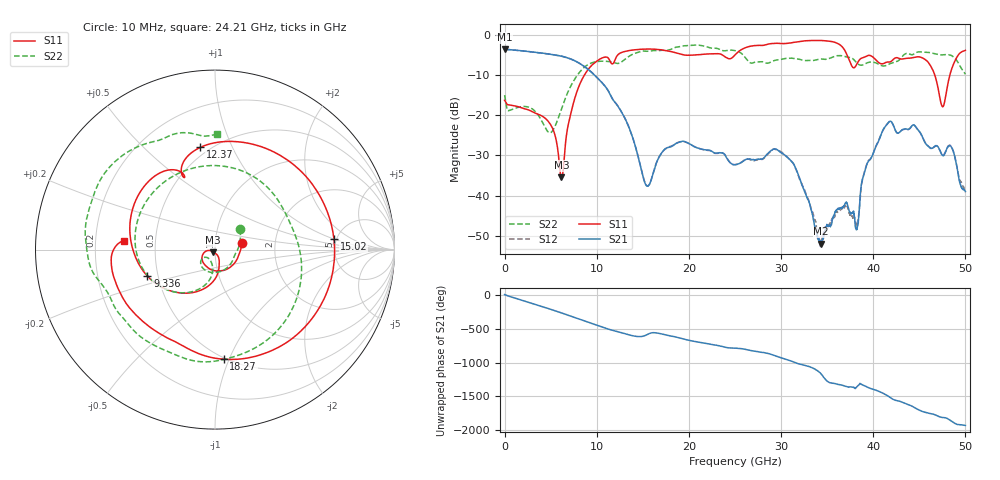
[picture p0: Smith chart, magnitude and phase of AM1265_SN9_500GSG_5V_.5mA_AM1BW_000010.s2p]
!Keysight Technologies,N5245B,MY58422270,A.16.20.02
!Date: Thursday, March 05, 2026 00:26:45
!Correction: S11(C  2-Port  )
!S21(C  2-Port  )
!S12(C  2-Port  )
!S22(C  2-Port  )
!S2P File: Measurements: S11, S21, S12, S22:
# Hz S  dB  R 50
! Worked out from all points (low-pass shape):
!   3201 points, 10 MHz to 50 GHz, reference 50 ohm
!   highest |S21| = -3.57 dB at 10 MHz (marker M1); lowest = -52.0 dB at 34.36 GHz (marker M2)
!   |S21| within 3 dB of the highest: start of sweep to 7.746 GHz
!   lowest |S11| = -35.4 dB at 6.181 GHz (marker M3), VSWR 1.03, Z = 49 - j1.38 ohm
!   |S11| at or under -10 dB: start of sweep to 8.665 GHz; 46.68 GHz to 48.31 GHz (1.63 GHz wide, 3.43 % of centre)
!   |S22| runs from -24.4 to -2.5 dB; largest |S21 - S12| = 0.011
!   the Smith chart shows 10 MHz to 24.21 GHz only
!   S11 on the Smith chart (normalised r, x): 10 MHz: 1.35, +0.11; 9.336 GHz: 0.44, -0.15; 12.37 GHz: 0.45, +0.76; 15.02 GHz: 4.75, +1.02; 18.27 GHz: 0.49, -0.96; 24.21 GHz: 0.32, +0.04
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1e7  -16.26 14.4  -3.57 4.0  -3.60 3.5  -14.99 39.0
2.322038e9  -18.46 -86.1  -4.06 -98.8  -4.06 -98.8  -17.83 -107.5
4.212284e9  -20.39 -135.9  -4.56 -179.3  -4.56 -179.3  -22.20 -145.0
6.180641e9  -35.43 -123.9  -5.29 92.9  -5.30 93.0  -18.45 -96.3
8.352081e9  -11.34 -117.8  -7.38 -10.1  -7.38 -10.0  -8.74 -145.5
9.336259e9  -7.86 -158.5  -9.08 -56.7  -9.06 -56.6  -7.07 178.2
1.107029e10  -5.52 129.4  -13.26 -136.4  -13.26 -136.4  -6.57 97.6
1.23669e10  -4.80 98.2  -17.95 173.1  -17.95 173.1  -7.09 22.5
1.502262e10  -3.54 5.2  -35.25 108.7  -35.11 108.6  -4.00 -99.9
1.667854e10  -3.62 -44.5  -30.79 153.3  -30.76 153.8  -3.91 -141.1
1.827197e10  -4.26 -85.4  -27.54 106.5  -27.49 106.5  -3.37 -166.7
2.420828e10  -5.82 174.5  -31.02 -60.7  -30.94 -60.2  -3.84 88.8
2.5005e10  -4.99 174.1  -32.29 -67.0  -32.27 -66.9  -3.91 70.9
2.95041e10  -2.08 96.1  -28.45 173.6  -28.56 173.4  -6.25 -19.7
3.334708e10  -1.39 35.6  -44.28 5.0  -43.85 5.9  -6.35 -127.1
3.43625e10  -1.39 17.9  -51.97 -90.6  -51.68 119.2  -6.00 -148.4
3.673703e10  -3.24 -32.4  -42.77 102.6  -42.77 103.0  -5.25 165.1
3.823673e10  -7.21 -22.0  -48.24 84.4  -47.42 12.5  -7.01 138.1
4.167354e10  -6.74 -54.1  -21.75 -59.5  -21.69 -60.0  -7.29 116.7
4.509473e10  -5.51 -101.5  -24.30 92.7  -24.32 93.3  -4.21 75.7
4.770358e10  -17.08 68.5  -29.87 -11.2  -29.66 -11.4  -4.91 39.1
5e10  -3.85 -72.5  -38.96 -127.7  -39.18 -126.7  -9.77 3.4
